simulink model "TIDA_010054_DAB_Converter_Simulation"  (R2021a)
settings: Solver=ode23tb  StartTime=0.0  StopTime=t_sim  RelTol=1e-3
undefined symbols (not defined in the file or in its folder): plecs

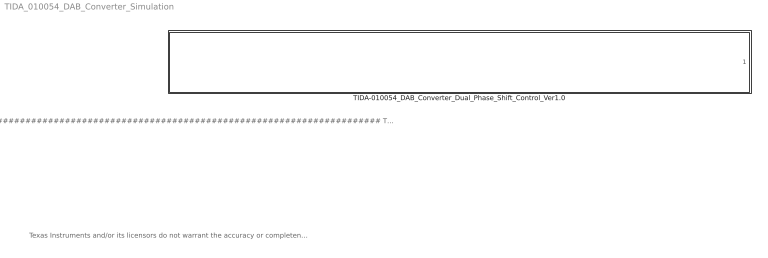
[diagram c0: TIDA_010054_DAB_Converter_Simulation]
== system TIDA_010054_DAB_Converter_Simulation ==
  note: ############################################################################# TI Release: TIDA_010054_DAB_Converter_Single_Phase_Shift_Control_Ver1.0 Release Date: Sep 28 2022 Copyright: Copyright (C) 2022 Texas Instruments Incorporated - http://www.ti.com/ ALL RIGHTS RESERVED #############################################################################
  note: Texas Instruments and/or its licensors do not warrant the accuracy or completeness of this specification or any information contained therein. Texas Instruments and/or its licensors do not warrant that this design will meet the specifications, will be suitable for your application or fit for any particular purpose, or will operate in an implementation. Texas Instruments and/or its licensors do not warrant that the design is production worthy. You should completely validate and test your design implementation to confirm the system functionality for your application.
  TIDA-010054_DAB_Converter_Dual_Phase_Shift_Control_Ver1.0 : Subsystem  LoadFcn=plecs('sl', 200);  InitFcn=plecs('sl', 214);  StartFcn=plecs('sl', 208);  StopFcn=plecs('sl', 209);  mask(PlecsCircuit){PLECSData=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}
      mask prompts: PLECSData "PLECS Data (Do not delete or modify!)"
      mask init:
      | % PLACE CUSTOM INITIALIZATIONS ABOVE
      | % DO NOT REMOVE
      | plecs('sl', 215);
      | % DO NOT REMOVE

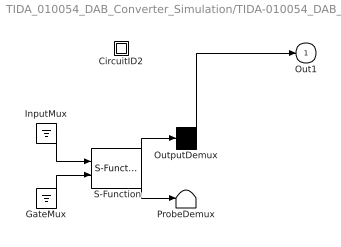
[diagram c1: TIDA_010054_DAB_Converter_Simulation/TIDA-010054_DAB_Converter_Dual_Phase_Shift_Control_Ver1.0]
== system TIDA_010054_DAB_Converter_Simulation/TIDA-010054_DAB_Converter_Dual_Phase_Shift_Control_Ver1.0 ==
  " CircuitID2 " : Subsystem
  " GateMux " : Ground
  " InputMux " : Ground
  " OutputDemux " : Demux  Outputs=[ 14 ]
  " ProbeDemux " : Terminator
  " S-Function " : S-Function  FunctionName=plecs  SFunctionDeploymentMode=off  EnableBusSupport=off
  Out1 : Outport  PortDimensions=14
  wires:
  " InputMux "/1 -> " S-Function "/1
  " GateMux "/1 -> " S-Function "/2
  " S-Function "/1 -> " OutputDemux "/1
  " S-Function "/2 -> " ProbeDemux "/1
  " OutputDemux "/1 -> Out1/1

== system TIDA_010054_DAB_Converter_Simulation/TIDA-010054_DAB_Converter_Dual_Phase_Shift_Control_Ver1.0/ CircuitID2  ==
